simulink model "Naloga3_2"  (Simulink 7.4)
settings: Solver=ode45  StartTime=0.0  StopTime=10.0  RelTol=1e-3
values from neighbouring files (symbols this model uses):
  b = 3*d    [fun.m]
undefined symbols (not defined in the file or in its folder): A

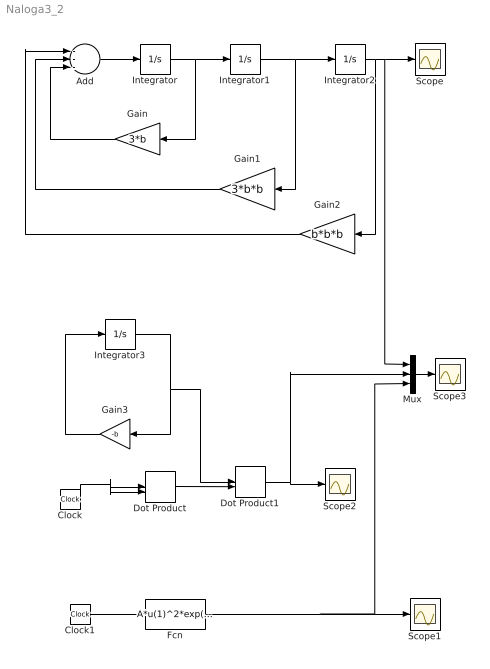
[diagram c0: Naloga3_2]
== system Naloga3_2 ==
  Add : Sum  Inputs=---  OutDataType=sfix(16)  OutScaling=2^-10
  Clock : Clock
  Clock1 : Clock
  Dot Product : DotProduct  OutDataType=sfix(16)  OutScaling=2^-10
  Dot Product1 : DotProduct  OutDataType=sfix(16)  OutScaling=2^-10
  Fcn : Fcn  Expr=A*u(1)^2*exp(-b*u(1))
  Gain : Gain  Gain=3*b  ParameterDataType=sfix(16)  ParameterScaling=2^0  OutDataType=sfix(16)  OutScaling=2^0
  Gain1 : Gain  Gain=3*b*b  ParameterDataType=sfix(16)  ParameterScaling=2^0  OutDataType=sfix(16)  OutScaling=2^0
  Gain2 : Gain  Gain=b*b*b  ParameterDataType=sfix(16)  ParameterScaling=2^0  OutDataType=sfix(16)  OutScaling=2^0
  Gain3 : Gain  Gain=-b  ParameterDataType=sfix(16)  ParameterScaling=2^0  OutDataType=sfix(16)  OutScaling=2^0
  Integrator : Integrator  InitialCondition=2*A
  Integrator1 : Integrator
  Integrator2 : Integrator
  Integrator3 : Integrator  InitialCondition=1
  Mux : Mux  Inputs=3
  Scope{,1..3} (4 alike) : Scope
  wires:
  Add/1 -> Integrator/1
  Integrator/1 -> Integrator1/1, Gain/1
  Integrator1/1 -> Integrator2/1, Gain1/1
  Gain/1 -> Add/3
  Gain1/1 -> Add/2
  Integrator2/1 -> Gain2/1, Scope/1, Mux/1
  Gain2/1 -> Add/1
  Integrator3/1 -> Gain3/1, Dot Product1/1
  Gain3/1 -> Integrator3/1
  Clock/1 -> Dot Product/1, Dot Product/2
  Dot Product/1 -> Dot Product1/2
  Dot Product1/1 -> Scope2/1, Mux/2
  Clock1/1 -> Fcn/1
  Fcn/1 -> Scope1/1, Mux/3
  Mux/1 -> Scope3/1
